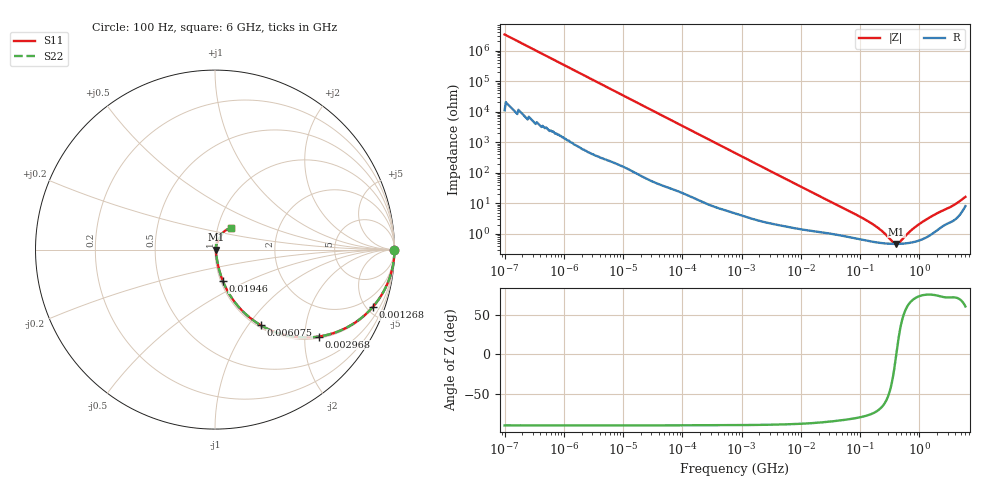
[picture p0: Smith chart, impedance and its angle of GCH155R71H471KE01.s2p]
!Murata Part Number: GCH155R71H471KE01
!These Parameters are Measured in Series Mode Connection
!Data Generated on Mar 13, 2026
!  o--ll--o
!Port1  Port2
!  o------o
!Operation Temp=25[degC], DC Bias Voltage=0[V]
!Freq. Start=100[Hz] Stop=6[GHz] 401[Steps]
# Hz S RI R 50
!Freq.(Hz) S11(Real) S11(Imag) S21(Real) S21(Imag) S12(Real) S12(Imag) S22(Real) S22(Imag)
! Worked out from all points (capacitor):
!   401 points, 100 Hz to 6 GHz, reference 50 ohm
!   read as one part in series: C = 473 pF near 109 Hz
!   lowest |Z| = 471 mohm at 408.7 MHz (marker M1)
!   series resonance near 409.5 MHz, so ESL is about 320 pH
!   S11 on the Smith chart (normalised r, x): 100 Hz: open; 1.268 MHz: 1.07, -5.46; 2.968 MHz: 1.04, -2.35; 6.075 MHz: 1.03, -1.15; 19.46 MHz: 1.02, -0.37; 6 GHz: 1.16, +0.28
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100  1 -2.98e-05  1e-07 2.98e-05  1e-07 2.98e-05  1 -2.98e-05
350  1 -0.000104  5e-07 0.000104  5e-07 0.000104  1 -0.000104
2008  1 -0.000593  2.5e-06 0.000593  2.5e-06 0.000593  1 -0.000593
40335  0.9998 -0.0118  0.000199 0.0118  0.000199 0.0118  0.9998 -0.0118
241822  0.9946 -0.0699  0.00542 0.0699  0.00542 0.0699  0.9946 -0.0699
774597  0.9501 -0.2126  0.0499 0.2126  0.0499 0.2126  0.9501 -0.2126
1267578  0.8788 -0.3201  0.1212 0.3201  0.1212 0.3201  0.8788 -0.3201
2967816  0.5777 -0.4845  0.4223 0.4845  0.4223 0.4845  0.5777 -0.4845
6075234  0.2559 -0.4219  0.7441 0.4219  0.7441 0.4219  0.2559 -0.4219
9506416  0.1301 -0.3175  0.8699 0.3175  0.8699 0.3175  0.1301 -0.3175
1.555665e7  0.0599 -0.2115  0.9401 0.2115  0.9401 0.2115  0.0599 -0.2115
1.946e7  0.0428 -0.1729  0.9572 0.1729  0.9572 0.1729  0.0428 -0.1729
4.556224e7  0.0151 -0.0777  0.9849 0.0777  0.9849 0.0777  0.0151 -0.0777
1.395531e8  0.00642 -0.0244  0.9936 0.0244  0.9936 0.0244  0.00642 -0.0244
2.183701e8  0.00523 -0.0129  0.9948 0.0129  0.9948 0.0129  0.00523 -0.0129
3.124326e8  0.00478 -0.00531  0.9952 0.00531  0.9952 0.00531  0.00478 -0.00531
3.737127e8  0.0047 -0.00178  0.9953 0.00178  0.9953 0.00178  0.0047 -0.00178
4.087225e8  0.00469 -3.73e-05  0.9953 3.73e-05  0.9953 3.73e-05  0.00469 -3.73e-05
4.674818e8  0.00473 0.00259  0.9953 -0.00259  0.9953 -0.00259  0.00473 0.00259
7.31507e8  0.00533 0.012  0.9947 -0.012  0.9947 -0.012  0.00533 0.012
1.144649e9  0.00729 0.0239  0.9927 -0.0239  0.9927 -0.0239  0.00729 0.0239
6e9  0.0907 0.1192  0.9093 -0.1192  0.9093 -0.1192  0.0907 0.1192
